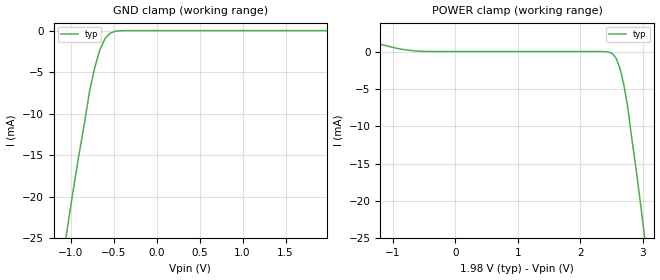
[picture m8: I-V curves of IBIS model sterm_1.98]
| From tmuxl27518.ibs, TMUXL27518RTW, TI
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| sterm_1.98
[Model]   sterm_1.98
Model_type   Terminator
|   typ   min   max
C_comp   4.014581e-12   NA   NA
[Voltage Range]   1.98   NA   NA
[Temperature Range]   27   NA   NA
[Power Clamp Reference]   1.98   NA   NA
[GND Clamp Reference]   0   NA   NA
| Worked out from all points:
|   GND clamp passes 1 mA (typ) near -0.60 V on its own axis
|   POWER clamp passes 1 mA (typ) near -1.21 V on its own axis
[GND Clamp]
|   Voltage   I(typ)   I(min)   I(max)
-3.96V    -335.1mA   NA         NA
-1.08V    -26.62mA   NA         NA
-1.02V    -22.48mA   NA         NA
-960mV    -18.5mA    NA         NA
-840mV    -11.13mA   NA         NA
-780mV    -7.255mA   NA         NA
-720mV    -4.428mA   NA         NA
-660mV    -2.296mA   NA         NA
-600mV    -948uA     NA         NA
-540mV    -300.9uA   NA         NA
-360mV    -2.72uA    NA         NA
1.98V     315.8pA    NA         NA
[POWER Clamp]
|   Voltage   I(typ)   I(min)   I(max)
-1.98V    2.91mA     NA         NA
-1.14V    838.7uA    NA         NA
-660mV    97.89uA    NA         NA
2.34V     -2.72uA    NA         NA
2.52V     -300.9uA   NA         NA
2.58V     -948uA     NA         NA
2.64V     -2.296mA   NA         NA
2.7V      -4.428mA   NA         NA
2.76V     -7.255mA   NA         NA
3V        -22.48mA   NA         NA
3.06V     -26.62mA   NA         NA
3.96V     -106.8mA   NA         NA
